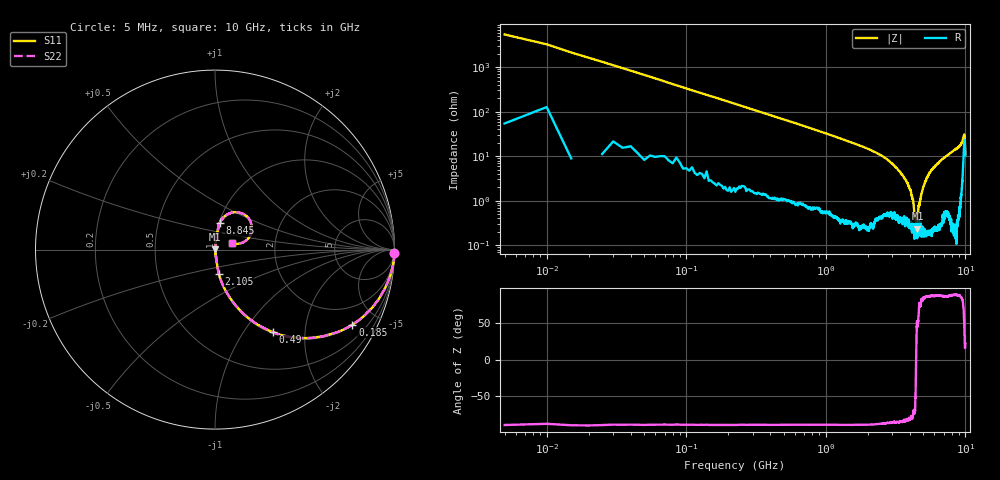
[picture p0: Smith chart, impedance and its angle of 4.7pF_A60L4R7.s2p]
! Amotech Co.,Ltd.
! http://www.amotech.co.kr/
! Part Number: A60L4R7
! These Parameters are Measured in Series Mode Connection
! Operation Temp=25[degC], DC Bias Voltage=0[V]
! Freq. Start=5[MHz] Stop=10[GHz], 2000[Steps]
! Date: Monday, July 14, 2020, 09:31:50
# GHZ S RI R 50.000000
!Freq.(Hz) S11(Real) S11(Imag) S21(Real) S21(Imag) S12(Real) S12(Imag) S22(Real) S22(Imag)
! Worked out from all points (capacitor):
!   2000 points, 5 MHz to 10 GHz, reference 50 ohm
!   read as one part in series: C = 4.77 pF near 55 MHz
!   lowest |Z| = 236 mohm at 4.53 GHz (marker M1)
!   series resonance near 4.438 GHz, so ESL is about 270 pH
!   S11 on the Smith chart (normalised r, x): 5 MHz: open; 185 MHz: 1.04, -3.64; 490 MHz: 1.02, -1.37; 2.105 GHz: 1.01, -0.27; 8.845 GHz: 1.01, +0.31; 10 GHz: 1.21, +0.08
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0.005  0.9995 -0.0184  0.000524 0.0184  0.000524 0.0184  0.9995 -0.0184
0.08  0.9423 -0.225  0.0577 0.225  0.0577 0.225  0.9423 -0.225
0.185  0.7658 -0.4184  0.2342 0.4184  0.2342 0.4184  0.7658 -0.4184
0.49  0.3215 -0.4596  0.6785 0.4596  0.6785 0.4596  0.3215 -0.4596
0.915  0.1174 -0.3139  0.8826 0.3139  0.8826 0.3139  0.1174 -0.3139
1.675  0.0354 -0.1764  0.9646 0.1764  0.9646 0.1764  0.0354 -0.1764
2.105  0.0212 -0.1335  0.9788 0.1335  0.9788 0.1335  0.0212 -0.1335
3.34  0.00575 -0.0462  0.9942 0.0462  0.9942 0.0462  0.00575 -0.0462
4.055  0.00348 -0.0161  0.9965 0.0161  0.9965 0.0161  0.00348 -0.0161
4.22  0.00282 -0.0101  0.9972 0.0101  0.9972 0.0101  0.00282 -0.0101
4.47  0.00257 0.00181  0.9974 -0.00181  0.9974 -0.00181  0.00257 0.00181
4.53  0.00166 0.00167  0.9983 -0.00167  0.9983 -0.00167  0.00166 0.00167
4.645  0.00264 0.00698  0.9974 -0.00698  0.9974 -0.00698  0.00264 0.00698
5.005  0.00207 0.0204  0.9979 -0.0204  0.9979 -0.0204  0.00207 0.0204
5.72  0.00407 0.0494  0.9959 -0.0494  0.9959 -0.0494  0.00407 0.0494
6.67  0.00918 0.0788  0.9908 -0.0788  0.9908 -0.0788  0.00918 0.0788
8.335  0.0202 0.1335  0.9798 -0.1335  0.9798 -0.1335  0.0202 0.1335
8.845  0.0265 0.1493  0.9735 -0.1493  0.9735 -0.1493  0.0265 0.1493
9.485  0.0648 0.1929  0.9352 -0.1929  0.9352 -0.1929  0.0648 0.1929
9.775  0.182 0.1807  0.818 -0.1807  0.818 -0.1807  0.182 0.1807
9.865  0.2005 0.0881  0.7995 -0.0881  0.7995 -0.0881  0.2005 0.0881
10  0.0957 0.0345  0.9043 -0.0345  0.9043 -0.0345  0.0957 0.0345
